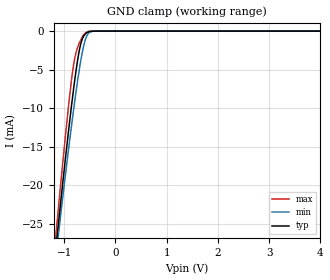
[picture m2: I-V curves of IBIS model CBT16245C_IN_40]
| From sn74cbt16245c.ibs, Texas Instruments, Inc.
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[Model]   CBT16245C_IN_40
Model_type  Input
Vinl=0.8
Vinh=2
| variable   typ   min   max
C_comp   2.54pF   1.92pF   3.25pF
[Temperature Range]   40   100   -40
| Ambient temperature   25   85   -40
[Voltage range]   4   4   4
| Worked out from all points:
|   GND clamp passes 1 mA (typ) near -0.64 V on its own axis
[GND Clamp]
| CBT16245C_IN_40
|   Voltage   I(typ)   I(min)   I(max)
-5V       -302.2mA   -280.5mA   -327.4mA
-1.145V   -27.15mA   -28.38mA   -25.39mA
-1.11V    -24.93mA   -26.36mA   -22.92mA
-1.08V    -23.05mA   -24.64mA   -20.82mA
-925mV    -13.66mA   -15.99mA   -10.47mA
-815mV    -7.538mA   -10.24mA   -4.411mA
-765mV    -5.061mA   -7.792mA   -2.746mA
-685mV    -1.948mA   -4.262mA   -1.277mA
-610mV    -564.6uA   -1.706mA   -431.8uA
-550mV    -185.6uA   -539uA     -116.2uA
-410mV    -6.4uA     -14.18uA   -1.367uA
4V        94.32pA    243.3pA    55.56pA
